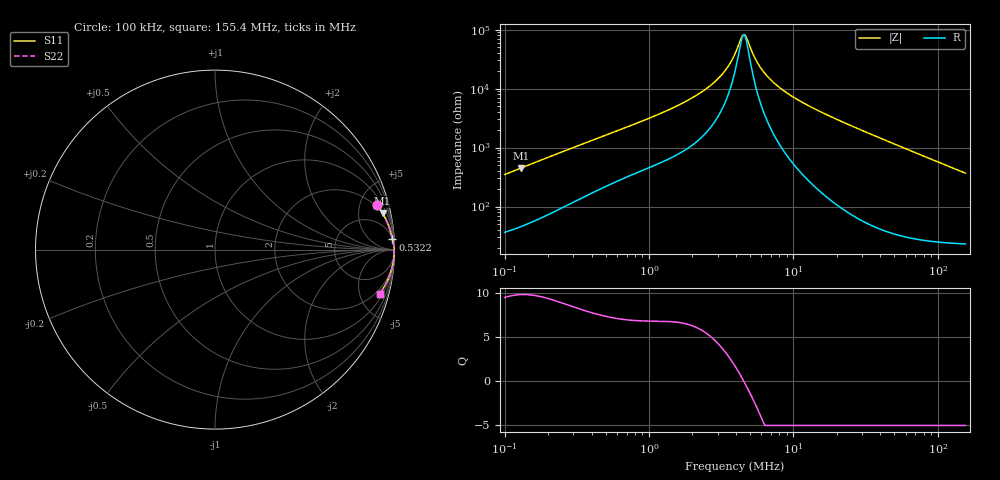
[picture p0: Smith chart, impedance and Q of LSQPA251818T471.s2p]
! LSQPA251818T471  S-PARAMETER MODEL  ( General Type )
! Model Generated by TAIYO YUDEN Corporation (http://www.ty-top.com)
! Version 3.0
! TAIYO YUDEN Control No. 160907NF25SB-FAC
! Copyright(c) 2007 TAIYO YUDEN CO.,LTD. All Rights Reserved.
! Product Description (link to TY-COMPAS)
! https://ds.yuden.co.jp/TYCOMPAS/or/detail?pn=LSQPA251818T471K&u=M
! Products Name : Inductors
! Characteristics :
!  Inductance : 470 uH , SRF(min) : 3.5 MHz , DC Resistance(max) : 28.6 Ohm
!  Rated Current : Saturation :80 mA , Temp Rise : 70 mA (40 degC)
!  Case Size : 2.5 x 1.8 / 0.098 x 0.071 [mm/inch] , Thickness : 1.8 / 0.071 [mm/inch]
!  (Conditions: Temperature = 25 degC , DC Bias Current/Voltage = 0A / 0V)
! External Node Assignments :
!  1  o---GGG---o  2
! GND o---------o GND
! Frequency Range : 0.1MHz  -  155.401204MHz  [ 402 STEP ]
# MHz S RI R 50
! Freq[MHz].  S11 Real  S11 Imag  S21 Real  S21 Imag  S12 Real  S12 Imag  S22 Real  S22 Imag
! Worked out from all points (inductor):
!   401 points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, 100 kHz to 155.4 MHz, reference 50 ohm
!   read as one part in series: L = 549 uH near 103.7 kHz
!   highest Q = 9.8 at 129.3 kHz (marker M1), where L = 549 uH
!   self-resonance near 4.483 MHz
!   S11 on the Smith chart (normalised r, x): 100 kHz: 1.73, +6.93; 532.2 kHz: 6, +34; 155.4 MHz: 1.46, -7.35
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0.1  0.9016 0.2497  0.0984 -0.2497  0.0984 -0.2497  0.9016 0.2497
0.12933  0.9339 0.2026  0.0661 -0.2026  0.0661 -0.2026  0.9339 0.2026
0.342427  0.982 0.0847  0.018 -0.0847  0.018 -0.0847  0.982 0.0847
0.532177  0.9889 0.0566  0.0111 -0.0566  0.0111 -0.0566  0.9889 0.0566
1.172566  0.9954 0.0266  0.00464 -0.0266  0.00464 -0.0266  0.9954 0.0266
1.890522  0.9974 0.0152  0.00261 -0.0152  0.00261 -0.0152  0.9974 0.0152
2.631463  0.9982 0.00889  0.00181 -0.00889  0.00181 -0.00889  0.9982 0.00889
2.992593  0.9984 0.00668  0.0016 -0.00668  0.0016 -0.00668  0.9984 0.00668
3.341331  0.9985 0.00486  0.00146 -0.00486  0.00146 -0.00486  0.9985 0.00486
3.662795  0.9986 0.00338  0.00136 -0.00338  0.00136 -0.00338  0.9986 0.00338
3.942096  0.9987 0.00221  0.0013 -0.00221  0.0013 -0.00221  0.9987 0.00221
4.401483  0.9988 0.000475  0.00122 -0.000475  0.00122 -0.000475  0.9988 0.000475
4.566214  0.9988 -0.000103  0.0012 0.000103  0.0012 0.000103  0.9988 -0.000103
4.650878  0.9988 -0.000393  0.00119 0.000393  0.00119 0.000393  0.9988 -0.000393
5.588835  0.9989 -0.00332  0.00112 0.00332  0.00112 0.00332  0.9989 -0.00332
6.126528  0.9989 -0.00482  0.00111 0.00482  0.00111 0.00482  0.9989 -0.00482
6.715953  0.9989 -0.00636  0.0011 0.00636  0.0011 0.00636  0.9989 -0.00636
8.84682  0.9988 -0.0114  0.00115 0.0114  0.00115 0.0114  0.9988 -0.0114
13.49882  0.9985 -0.0209  0.00149 0.0209  0.00149 0.0209  0.9985 -0.0209
46.22367  0.9913 -0.0793  0.00867 0.0793  0.00867 0.0793  0.9913 -0.0793
92.90788  0.9682 -0.156  0.0318 0.156  0.0318 0.156  0.9682 -0.156
155.4012  0.918 -0.2446  0.082 0.2446  0.082 0.2446  0.918 -0.2446
